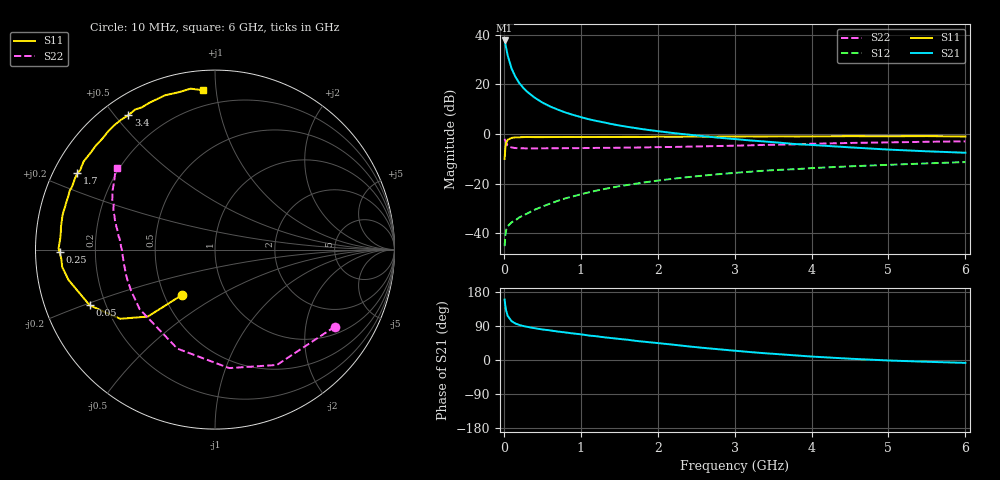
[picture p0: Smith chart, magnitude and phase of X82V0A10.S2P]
! SIEMENS Small Signal Semiconductors
! BFP136W
! Si NPN RF Bipolar Junction Transistor in SOT343
! VCE = 2 V  IC = 100 mA
! Common Emitter S-Parameters:  September  1994
# GHz  S  MA  R  50
!  f  S11  S21  S12  S22
! GHz  MAG  ANG  MAG  ANG  MAG  ANG  MAG  ANG
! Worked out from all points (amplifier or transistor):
!   40 points, 10 MHz to 6 GHz, reference 50 ohm
!   highest |S21| = 37.7 dB at 10 MHz (marker M1)
!   |S21| within 3 dB of that: start of sweep to 29.99 MHz
!   unconditionally stable (mu >= 1): 451.2 MHz to 2.866 GHz
!   at 200 MHz: K = 0.72, MSG = 27.1 dB, |S12| = -33.6 dB
!   at 1.5 GHz: K = 1.11, MAG = 10.2 dB, |S12| = -21.1 dB
!   at 6 GHz: K = 0.98, MSG = 1.9 dB, |S12| = -11.3 dB
!   S11 on the Smith chart (normalised r, x): 10 MHz: 0.61, -0.35; 50 MHz: 0.14, -0.21; 250 MHz: 0.07, -0.01; 1.7 GHz: 0.07, +0.26; 3.4 GHz: 0.07, +0.54; 6 GHz: 0.11, +0.92
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0.01  0.315 -126.2  76.56 159.3  0.0055 67.3  0.7941 -32.7
0.02  0.5288 -135.1  64.98 142.4  0.009 54.8  0.7293 -61.8
0.03  0.6542 -143.9  54.2 130.5  0.0116 47.7  0.6649 -83.2
0.05  0.7639 -156.0  38.2 116.6  0.0139 38.3  0.59 -110.9
0.1  0.8335 -168.3  20.93 102.5  0.0166 35.9  0.5352 -141.6
0.15  0.8569 -173.5  14.2 96.4  0.0182 39.5  0.5206 -153.9
0.2  0.8575 -176.4  10.65 92.6  0.0208 43.2  0.5164 -160.6
0.25  0.8656 -179.0  8.59 89.8  0.0228 46.5  0.5151 -164.8
0.3  0.8715 179.5  7.181 87.7  0.0248 49.2  0.513 -167.6
0.4  0.8647 176.1  5.405 83.9  0.0298 53.8  0.5137 -171.4
0.5  0.8646 173.3  4.307 80.7  0.0345 57.8  0.5143 -174.0
0.6  0.8676 171.7  3.595 78.1  0.0395 59.8  0.5151 -175.7
0.7  0.8687 169.2  3.102 75.1  0.045 61.0  0.5161 -176.9
0.9  0.8703 165.8  2.425 70.1  0.0554 62.2  0.518 -179.5
1.1  0.8696 161.5  1.987 64.7  0.0665 62.4  0.5217 178.9
1.7  0.8764 151.0  1.324 50.9  0.0988 60.0  0.5335 174.0
2.2  0.8782 142.6  1.046 40.4  0.1254 55.9  0.5477 170.3
3.2  0.8927 125.8  0.742 21.0  0.1736 46.0  0.5911 161.4
3.4  0.8912 122.8  0.704 17.7  0.1831 43.8  0.6037 159.6
4.5  0.9037 107.9  0.538 3.4  0.2232 33.4  0.6599 149.8
5.5  0.9069 98.6  0.448 -4.7  0.2559 25.4  0.6971 143.1
6  0.8901 94.3  0.419 -7.6  0.2721 21.0  0.7112 140.1
